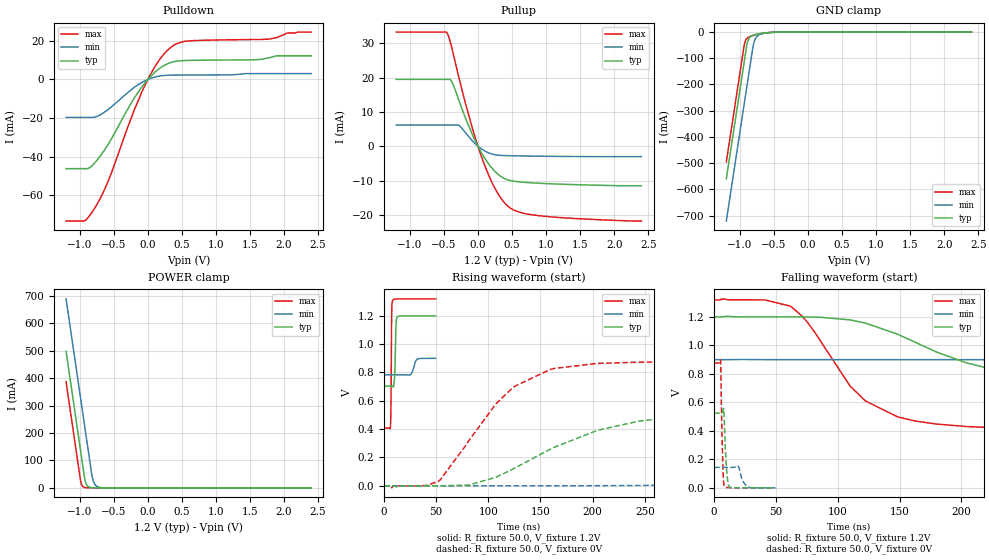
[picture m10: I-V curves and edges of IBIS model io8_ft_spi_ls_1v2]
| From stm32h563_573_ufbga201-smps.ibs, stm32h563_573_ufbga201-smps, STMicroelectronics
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[Model]   io8_ft_spi_ls_1v2
Model_type I/O
Polarity   Non-Inverting
Enable   Active-Low
| CAP_THRESHOLD on pad IOFT is "UDTCAPC" :
| Rising=20.0% of vddiom   Falling=80.0% of vddiom
| C_comp min and max val. don't necessarily correlate with the min and max pvt
| but are the smallest and greatest pad capacitance found.
| var   typ   min   max
C_comp   4.02950pF  3.92710pF  4.03445pF
|C_comp_pullup   2.45860pF  2.26995pF  2.18285pF
|C_comp_pulldown   1.57090pF  1.65715pF  1.85160pF
Vinl = 270.0mV
Vinh = 924.0mV
Vmeas = 600.0mV   | Reference voltage for timing measurements
Cref  = 50.0pF   | Timing specification test load capacitance value
Rref  = 100.0MOhm   | Timing specification test load resistance value
Vref  = 600.0mV   | Timing specification test load voltage
[Model Spec]
| TIME_THRESHOLD on pin ZIV11 is "CMOS" :
| Rising=40.0% of vdd   Falling=60.0% of vdd
Vinl 447.80000mV 344.80000mV 489.80000mV
Vinh 733.20000mV 535.20000mV 813.20000mV
| variable   typ   min   max
[Temperature Range] 25.0 125.0 -40.0
| variable   typ   min   max
[Voltage Range] 1.2V 900.0mV 1.32V
| variable   typ   min   max
[POWER Clamp Reference] 1.2V 900.0mV 1.32V
| variable   typ   min   max
[GND Clamp Reference] 0V 0V 0V
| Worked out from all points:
|   slope of the pulldown table from 0 to 0.18 V, typ, clamps not added: 30.6 ohm
|   slope of the pullup table from 0 to 0.18 V, typ, clamps not added: 31.3 ohm
|   GND clamp passes 1 mA (typ) near -0.52 V on its own axis
|   POWER clamp passes 1 mA (typ) near -0.84 V on its own axis
|   rising waveform, R_fixture 50.0, V_fixture 1.2V: 20-80 % time 1.02ns typ, 2.94ns min, 536ps max; typ from 0.704 V to 1.2 V
|   falling waveform, R_fixture 50.0, V_fixture 1.2V: 20-80 % time 102ns typ, 289ns min, 49.4ns max; typ from 1.2 V to 0.704 V
|   rising waveform, R_fixture 50.0, V_fixture 0V: 20-80 % time 102ns typ, 236ns min, 57.8ns max; typ from 0 V to 0.525 V
|   falling waveform, R_fixture 50.0, V_fixture 0V: 20-80 % time 1.86ns typ, 3.8ns min, 1.35ns max; typ from 0.525 V to 0 V
[POWER Clamp]
-1.2V     497.8mA    689.2mA    386.5mA
-990mV    140.8mA    332.2mA    29.53mA
-980mV    123.8mA    315.2mA    17.95mA
-960mV    89.81mA    281.2mA    6.634mA
-930mV    38.81mA    230.2mA    1.49mA
-900mV    12.07mA    179.2mA    334.8uA
-870mV    3.756mA    128.2mA    75.22uA
-820mV    536.4uA    44.98mA    6.246uA
-790mV    166.9uA    18.76mA    1.403uA
-750mV    35.18uA    5.846mA    191.9nA
-590mV    70.48nA    54.99uA    204.6pA
2.4V      0A         0A         0A
[GND Clamp]
-1.2V     -559.6mA   -720.6mA   -495.5mA
-940mV    -117.6mA   -278.6mA   -53.46mA
-930mV    -100.6mA   -261.6mA   -41.27mA
-900mV    -50.49mA   -210.6mA   -24.86mA
-880mV    -31.4mA    -176.6mA   -20.57mA
-850mV    -18.9mA    -125.6mA   -16.88mA
-810mV    -12.57mA   -58.3mA    -13.49mA
-780mV    -10.11mA   -29.57mA   -11.38mA
-740mV    -7.754mA   -14.31mA   -8.91mA
-640mV    -3.713mA   -4.821mA   -4.078mA
-390mV    -82.2uA    -288.6uA   -29.73uA
2.4V      3.859nA    727.3nA    172.3pA
| variable   typ   min   max
[Pullup Reference] 1.2V 900.0mV 1.32V
| variable   typ   min   max
[Pulldown Reference] 0V 0V 0V
[Pullup]
-1.2V     19.46mA    6.167mA    33.25mA
-450mV    19.46mA    6.167mA    32.87mA
-380mV    18.63mA    6.167mA    28.35mA
-280mV    13.4mA     6.087mA    20.06mA
-80mV     3.3mA      1.494mA    5.118mA
60mV      -2.179mA   -890.4uA   -3.476mA
260mV     -7.541mA   -2.511mA   -12.64mA
360mV     -9.094mA   -2.701mA   -15.73mA
460mV     -9.923mA   -2.763mA   -17.79mA
670mV     -10.5mA    -2.845mA   -19.55mA
920mV     -10.81mA   -2.911mA   -20.29mA
2.4V      -11.52mA   -3.044mA   -21.79mA
[Pulldown]
-1.2V     -46.17mA   -19.61mA   -73.27mA
-930mV    -46.17mA   -19.61mA   -73.17mA
-770mV    -42.8mA    -19.4mA    -66.04mA
-570mV    -32.88mA   -15.17mA   -51.58mA
-200mV    -9.658mA   -4.081mA   -15.89mA
-80mV     -3.488mA   -1.363mA   -5.887mA
130mV     4.529mA    1.468mA    8.049mA
340mV     8.782mA    2.249mA    16.66mA
540mV     9.805mA    2.304mA    19.74mA
1.79V     11.29mA    3.027mA    20.92mA
2.05V     12.25mA    3.027mA    24.04mA
2.4V      12.25mA    3.027mA    24.55mA
[Ramp]
dV/dt_r 315.13814mV/99.23117ns 86.03942mV/233.91033ns 525.77959mV/56.47325ns
dV/dt_f 297.80469mV/100.81045ns 69.85405mV/286.9225ns 547.13925mV/47.70979ns
R_load = 50.0
| Removed startup time: 0s 0s 0s  .
| Removed end time: 49.4ns.
[Rising Waveform]
R_fixture   = 50.0
V_fixture   = 1.2V
V_fixture_min = 900.0mV
V_fixture_max = 1.32V
0s        703.7mV    783.5mV    408.1mV
6.25ns    703.7mV    783.5mV    420.2mV
6.75ns    703.8mV    783.5mV    581.7mV
7.4ns     703.8mV    783.5mV    1.201V
8.05ns    702.3mV    783.5mV    1.304V
10.1ns    752.9mV    783.5mV    1.317V
11.65ns   1.148V     783.5mV    1.319V
13.1ns    1.195V     783.5mV    1.319V
32.3ns    1.2V       896.1mV    1.32V
49.4ns    1.2V       899.9mV    1.32V
| Removed startup time: 0s 0s 0s  .
| Removed end time: 1.9994us.
[Falling Waveform]
R_fixture   = 50.0
V_fixture   = 1.2V
V_fixture_min = 900.0mV
V_fixture_max = 1.32V
0s        1.2V       900mV      1.32V
61.2ns    1.2V       900mV      1.277V
75.3ns    1.2V       900mV      1.164V
122.4ns   1.157V     900mV      610.1mV
148.4ns   1.079V     900mV      498mV
204.1ns   877.5mV    899.9mV    430.6mV
285.7ns   758.9mV    898.1mV    411.9mV
445.9ns   710.4mV    871.8mV    408.2mV
856.9ns   703.7mV    794.6mV    408.1mV
1.999us   703.7mV    783.6mV    408.1mV
| Removed startup time: 0s 0s 0s  .
| Removed end time: 1.9994us.
[Rising Waveform]
R_fixture   = 50.0
V_fixture   = 0V
V_fixture_min = 0V
V_fixture_max = 0V
0s        166.5nV    851.1nV    114.4nV
52.1ns    -37.39uV   -10.39uV   30.81mV
81.6ns    5.815mV    -12.41uV   321.9mV
125.4ns   125.2mV    18.7uV     702.8mV
159.4ns   258.5mV    131.4uV    821.6mV
205ns     391.9mV    736.3uV    864mV
285.6ns   491.9mV    7.358mV    875.1mV
408.1ns   521.2mV    50.16mV    876.1mV
775.3ns   525.1mV    136.7mV    876.3mV
1.999us   525.2mV    143.4mV    876.3mV
| Removed startup time: 0s 0s 0s  .
| Removed end time: 49.4ns.
[Falling Waveform]
R_fixture   = 50.0
V_fixture   = 0V
V_fixture_min = 0V
V_fixture_max = 0V
0s        525.3mV    143.6mV    876.3mV
5.25ns    525.3mV    143.6mV    893.6mV
7.05ns    535.7mV    143.6mV    172.9mV
7.85ns    551.6mV    143.6mV    27.69mV
8.5ns     418.9mV    143.6mV    9.504mV
10ns      139.3mV    143.6mV    3.056mV
12.1ns    6.964mV    143.5mV    1.637mV
19.15ns   414.5uV    156.5mV    331.5uV
27.25ns   118.7uV    7.7mV      175.2uV
49.4ns    75.75uV    9.721uV    190.5uV
